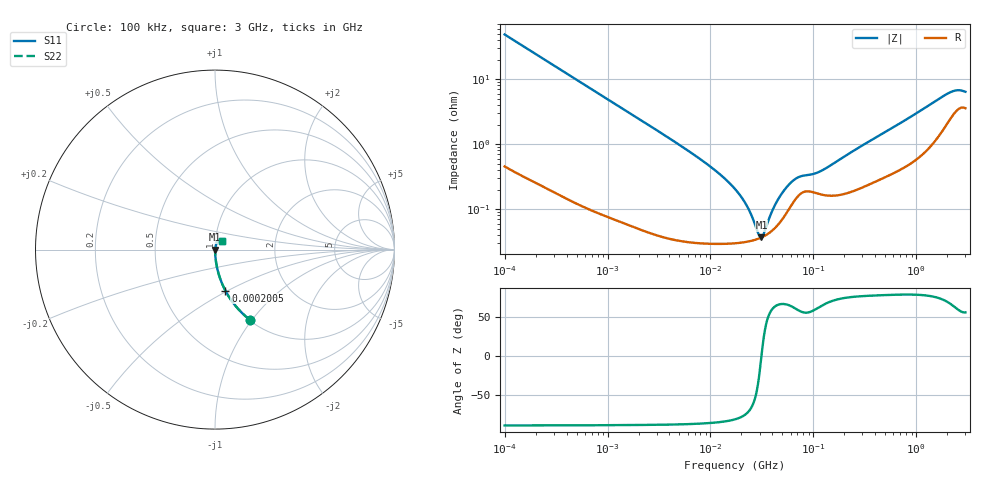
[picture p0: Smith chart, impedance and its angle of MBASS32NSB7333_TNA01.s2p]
! MBASS32NSB7333_TNA01  S-PARAMETER MODEL  ( Standard Model )
! Model Generated by TAIYO YUDEN Corporation (http://www.ty-top.com)
! Version 1.0
! TAIYO YUDEN Control No. 220601
! Copyright(c) 2013 TAIYO YUDEN CO.,LTD. All Rights Reserved.
! Product Description (link to TY-COMPAS)
! https://ds.yuden.co.jp/TYCOMPAS/or/detail?pn=MBASS32NSB7333KTNA01&u=M
! Products Name : Multilayer Ceramic Capacitors
! Characteristics :
!  Capacitance : 0.033 [uF] , Rated Voltage : 630 [V] , TCC : X7R
!  Case Size : 3.2 x 2.5 / 0.126 x 0.098 [mm/inch] , Thickness : 1.9 / 0.075 [mm/inch]
!  (Conditions: Temperature = 25 [degC] , DC Bias Voltage = 0 [V])
! External Node Assignments :
!  1  o---| |---o  2
! GND o---------o GND
! Frequency Range : 100kHz  -  3GHz  [ 401 STEP ]
# MHZ S RI R 50
! Freq[MHz].  S11 Real  S11 Imag  S21 Real  S21 Imag  S12 Real  S12 Imag  S22 Real  S22 Imag
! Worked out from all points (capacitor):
!   401 points, 100 kHz to 3 GHz, reference 50 ohm
!   read as one part in series: C = 32.6 nF near 105.3 kHz
!   lowest |Z| = 36.8 mohm at 31.33 MHz (marker M1)
!   series resonance near 31.31 MHz, so ESL is about 790 pH
!   S11 on the Smith chart (normalised r, x): 100 kHz: 1.01, -0.97; 200.5 kHz: 1.01, -0.49; 3 GHz: 1.07, +0.11
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0.1  0.1938 -0.3907  0.8062 0.3907  0.8062 0.3907  0.1938 -0.3907
0.200542  0.0582 -0.2289  0.9418 0.2289  0.9418 0.2289  0.0582 -0.2289
0.562235  0.00868 -0.0866  0.9913 0.0866  0.9913 0.0866  0.00868 -0.0866
3.161081  0.000629 -0.0156  0.9994 0.0156  0.9994 0.0156  0.000629 -0.0156
9.824692  0.000315 -0.0046  0.9997 0.0046  0.9997 0.0046  0.000315 -0.0046
13.7349  0.000302 -0.00296  0.9997 0.00296  0.9997 0.00296  0.000302 -0.00296
17.7727  0.000304 -0.00193  0.9997 0.00193  0.9997 0.00193  0.000304 -0.00193
22.41241  0.000316 -0.00111  0.9997 0.00111  0.9997 0.00111  0.000316 -0.00111
24.84619  0.000326 -0.000762  0.9997 0.000762  0.9997 0.000762  0.000326 -0.000762
29.00125  0.00035 -0.000253  0.9997 0.000253  0.9997 0.000253  0.00035 -0.000253
31.3325  0.000368 2.33e-06  0.9996 -2.33e-06  0.9996 -2.33e-06  0.000368 2.33e-06
32.98988  0.000383 0.000174  0.9996 -0.000174  0.9996 -0.000174  0.000383 0.000174
38.50681  0.000449 0.0007  0.9996 -0.0007  0.9996 -0.0007  0.000449 0.0007
42.68829  0.00052 0.00107  0.9995 -0.00107  0.9995 -0.00107  0.00052 0.00107
53.83243  0.000838 0.00192  0.9992 -0.00192  0.9992 -0.00192  0.000838 0.00192
69.65816  0.00154 0.00262  0.9985 -0.00262  0.9985 -0.00262  0.00154 0.00262
97.38194  0.00184 0.0029  0.9982 -0.0029  0.9982 -0.0029  0.00184 0.0029
129.3002  0.00165 0.00382  0.9983 -0.00382  0.9983 -0.00382  0.00165 0.00382
547.5153  0.00358 0.0163  0.9964 -0.0163  0.9964 -0.0163  0.00358 0.0163
2038.117  0.0242 0.054  0.9758 -0.054  0.9758 -0.054  0.0242 0.054
2441.062  0.0343 0.0553  0.9657 -0.0553  0.9657 -0.0553  0.0343 0.0553
3000  0.037 0.0493  0.963 -0.0493  0.963 -0.0493  0.037 0.0493
